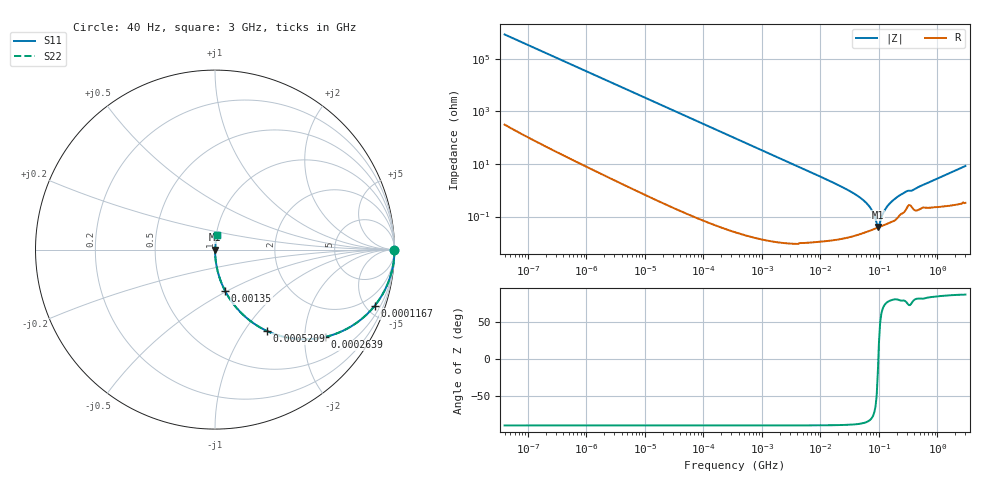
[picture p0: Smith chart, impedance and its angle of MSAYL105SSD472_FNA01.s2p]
! MSAYL105SSD472_FNA01  S-PARAMETER MODEL  ( General Type )
! Model Generated by TAIYO YUDEN Corporation (http://www.ty-top.com)
! Version 2.0
! TAIYO YUDEN Control No. 040624
! Copyright(c) 2004 TAIYO YUDEN CO.,LTD. All Rights Reserved.
! Product Description (link to TY-COMPAS)
! https://ds.yuden.co.jp/TYCOMPAS/or/detail?pn=MSAYL105SSD472KFNA01&u=M
! Products Name : Multilayer Ceramic Capacitors
! Characteristics :
!  Capacitance : 4700 pF , Rated Voltage : 10V
!  Case Size : 1.0 x 0.5 / 0.039 x 0.02 [mm/inch] , Thickness : 0.5 / 0.02 [mm/inch]
!  (Conditions: Temperature = 25 degC , DC Bias Current/Voltage = 0A / 0V)
! External Node Assignments :
!  1  o---| |---o  2
! GND o---------o GND
! Frequency Range : 40Hz  -  3GHz  [ 401 STEP ]
# MHz S RI R 50
! Freq[MHz].  S11 Real  S11 Imag  S21 Real  S21 Imag  S12 Real  S12 Imag  S22 Real  S22 Imag
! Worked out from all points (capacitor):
!   401 points, 40 Hz to 3 GHz, reference 50 ohm
!   read as one part in series: C = 4.82 nF near 44 Hz
!   lowest |Z| = 39.6 mohm at 95.69 MHz (marker M1)
!   series resonance near 97.49 MHz, so ESL is about 550 pH
!   S11 on the Smith chart (normalised r, x): 40 Hz: open; 116.7 kHz: 1.00, -5.66; 263.9 kHz: 1.00, -2.50; 520.9 kHz: 1.00, -1.27; 1.35 MHz: 1.00, -0.49; 3 GHz: 1.01, +0.17
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4e-05  1 -0.000121  6e-08 0.000121  6e-08 0.000121  1 -0.000121
0.000834  1 -0.00252  6.98e-06 0.00252  6.98e-06 0.00252  1 -0.00252
0.017386  0.9972 -0.0525  0.00277 0.0525  0.00277 0.0525  0.9972 -0.0525
0.04932  0.9782 -0.146  0.0218 0.146  0.0218 0.146  0.9782 -0.146
0.116704  0.889 -0.314  0.111 0.314  0.111 0.314  0.889 -0.314
0.263915  0.6105 -0.4875  0.3895 0.4875  0.3895 0.4875  0.6105 -0.4875
0.362475  0.4539 -0.4977  0.5461 0.4977  0.5461 0.4977  0.4539 -0.4977
0.52093  0.287 -0.4522  0.713 0.4522  0.713 0.4522  0.287 -0.4522
1.349647  0.0566 -0.2309  0.9434 0.2309  0.9434 0.2309  0.0566 -0.2309
7.222098  0.00217 -0.0454  0.9978 0.0454  0.9978 0.0454  0.00217 -0.0454
25.69909  0.00029 -0.0119  0.9997 0.0119  0.9997 0.0119  0.00029 -0.0119
48.47801  0.000242 -0.00507  0.9998 0.00507  0.9998 0.00507  0.000242 -0.00507
69.67004  0.000293 -0.00228  0.9997 0.00228  0.9997 0.00228  0.000293 -0.00228
79.8195  0.000324 -0.00133  0.9997 0.00133  0.9997 0.00133  0.000324 -0.00133
91.44753  0.000363 -0.000419  0.9996 0.000419  0.9996 0.000419  0.000363 -0.000419
95.68847  0.000378 -0.000119  0.9996 0.000119  0.9996 0.000119  0.000378 -0.000119
104.7695  0.00041 0.000476  0.9996 -0.000476  0.9996 -0.000476  0.00041 0.000476
125.5988  0.000487 0.00169  0.9995 -0.00169  0.9995 -0.00169  0.000487 0.00169
150.5692  0.000582 0.00296  0.9994 -0.00296  0.9994 -0.00296  0.000582 0.00296
284.0294  0.00178 0.00841  0.9982 -0.00841  0.9982 -0.00841  0.00178 0.00841
390.1008  0.00196 0.0102  0.998 -0.0102  0.998 -0.0102  0.00196 0.0102
3000  0.01 0.0818  0.99 -0.0818  0.99 -0.0818  0.01 0.0818
